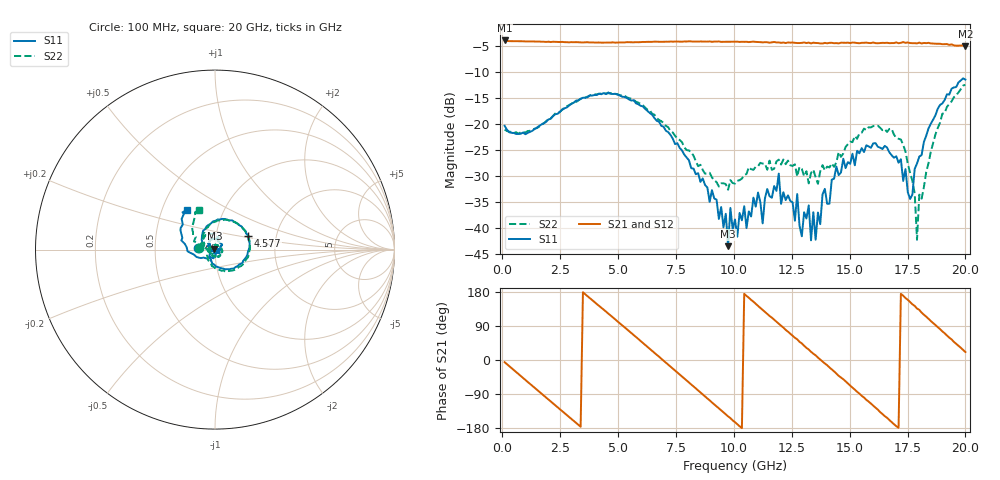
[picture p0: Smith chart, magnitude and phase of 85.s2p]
!Agilent Technologies,N5230C,MY49001569,A.09.33.09
!Agilent N5230C: A.09.33.09
!Date: Tuesday, July 28, 2015 10:21:08
!Correction: S11(Full 2 Port(1,2))
!S21(Full 2 Port(1,2))
!S12(Full 2 Port(1,2))
!S22(Full 2 Port(1,2))
!S2P File: Measurements: S11, S21, S12, S22:
# Hz S  dB  R 50
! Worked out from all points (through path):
!   201 points, 100 MHz to 20 GHz, reference 50 ohm
!   highest |S21| = -3.87 dB at 100 MHz (marker M1); lowest = -5.0 dB at 20 GHz (marker M2)
!   group delay of S21, straight-line fit = 147 ps
!   lowest |S11| = -43.5 dB at 9.752 GHz (marker M3), VSWR 1.01, Z = 49.6 + j0.565 ohm
!   |S11| at or under -10 dB: start of sweep to end of sweep
!   |S22| runs from -42.2 to -12.4 dB; largest |S21 - S12| = 0.023
!   S11 on the Smith chart (normalised r, x): 100 MHz: 0.82, +0.02; 4.577 GHz: 1.44, +0.23; 20 GHz: 0.67, +0.32
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1e8  -20.30 174.2  -3.87 -5.8  -3.86 -5.8  -21.05 172.4
1.7915e9  -19.82 135.5  -4.12 -94.0  -4.13 -94.0  -19.81 131.5
3.483e9  -14.91 71.4  -4.27 178.8  -4.28 178.6  -14.93 67.5
4.5775e9  -13.89 22.8  -4.29 122.5  -4.31 122.3  -14.05 18.7
6.7665e9  -19.51 -74.7  -4.13 8.9  -4.14 8.7  -19.18 -81.1
8.3585e9  -29.64 -153.2  -4.08 -75.0  -4.10 -75.4  -27.12 -156.5
9.7515e9  -43.49 121.7  -4.13 -148.8  -4.11 -148.5  -32.62 85.8
1.005e10  -38.34 65.9  -4.11 -164.2  -4.13 -164.6  -31.44 69.0
1.1045e10  -33.15 -3.8  -4.17 142.7  -4.15 143.6  -28.09 -3.6
1.1244e10  -39.09 -16.2  -4.24 132.5  -4.15 132.5  -27.58 -15.5
1.19405e10  -29.52 -42.0  -4.25 96.0  -4.22 95.5  -26.82 -54.1
1.29355e10  -41.58 -84.3  -4.34 43.7  -4.36 42.4  -28.61 -117.3
1.3433e10  -36.95 -103.2  -4.30 16.7  -4.50 16.3  -28.77 -141.7
1.35325e10  -42.24 -110.2  -4.36 12.3  -4.34 11.5  -30.22 -148.4
1.51245e10  -25.69 138.4  -4.28 -73.1  -4.41 -72.4  -23.46 150.3
1.67165e10  -25.41 71.4  -4.39 -158.4  -4.35 -158.6  -20.92 90.4
1.7413e10  -28.64 2.3  -4.33 163.5  -4.38 163.9  -25.27 70.1
1.7612e10  -34.39 -20.6  -4.37 153.0  -4.32 152.5  -29.35 68.9
1.79105e10  -27.57 -106.4  -4.44 135.9  -4.36 136.5  -42.25 106.9
1.801e10  -26.23 -98.9  -4.29 132.2  -4.48 130.4  -33.56 86.8
1.87065e10  -18.27 -167.5  -4.50 92.5  -4.50 92.3  -21.98 161.6
2e10  -11.40 125.3  -5.02 21.0  -5.10 20.0  -12.43 111.8
